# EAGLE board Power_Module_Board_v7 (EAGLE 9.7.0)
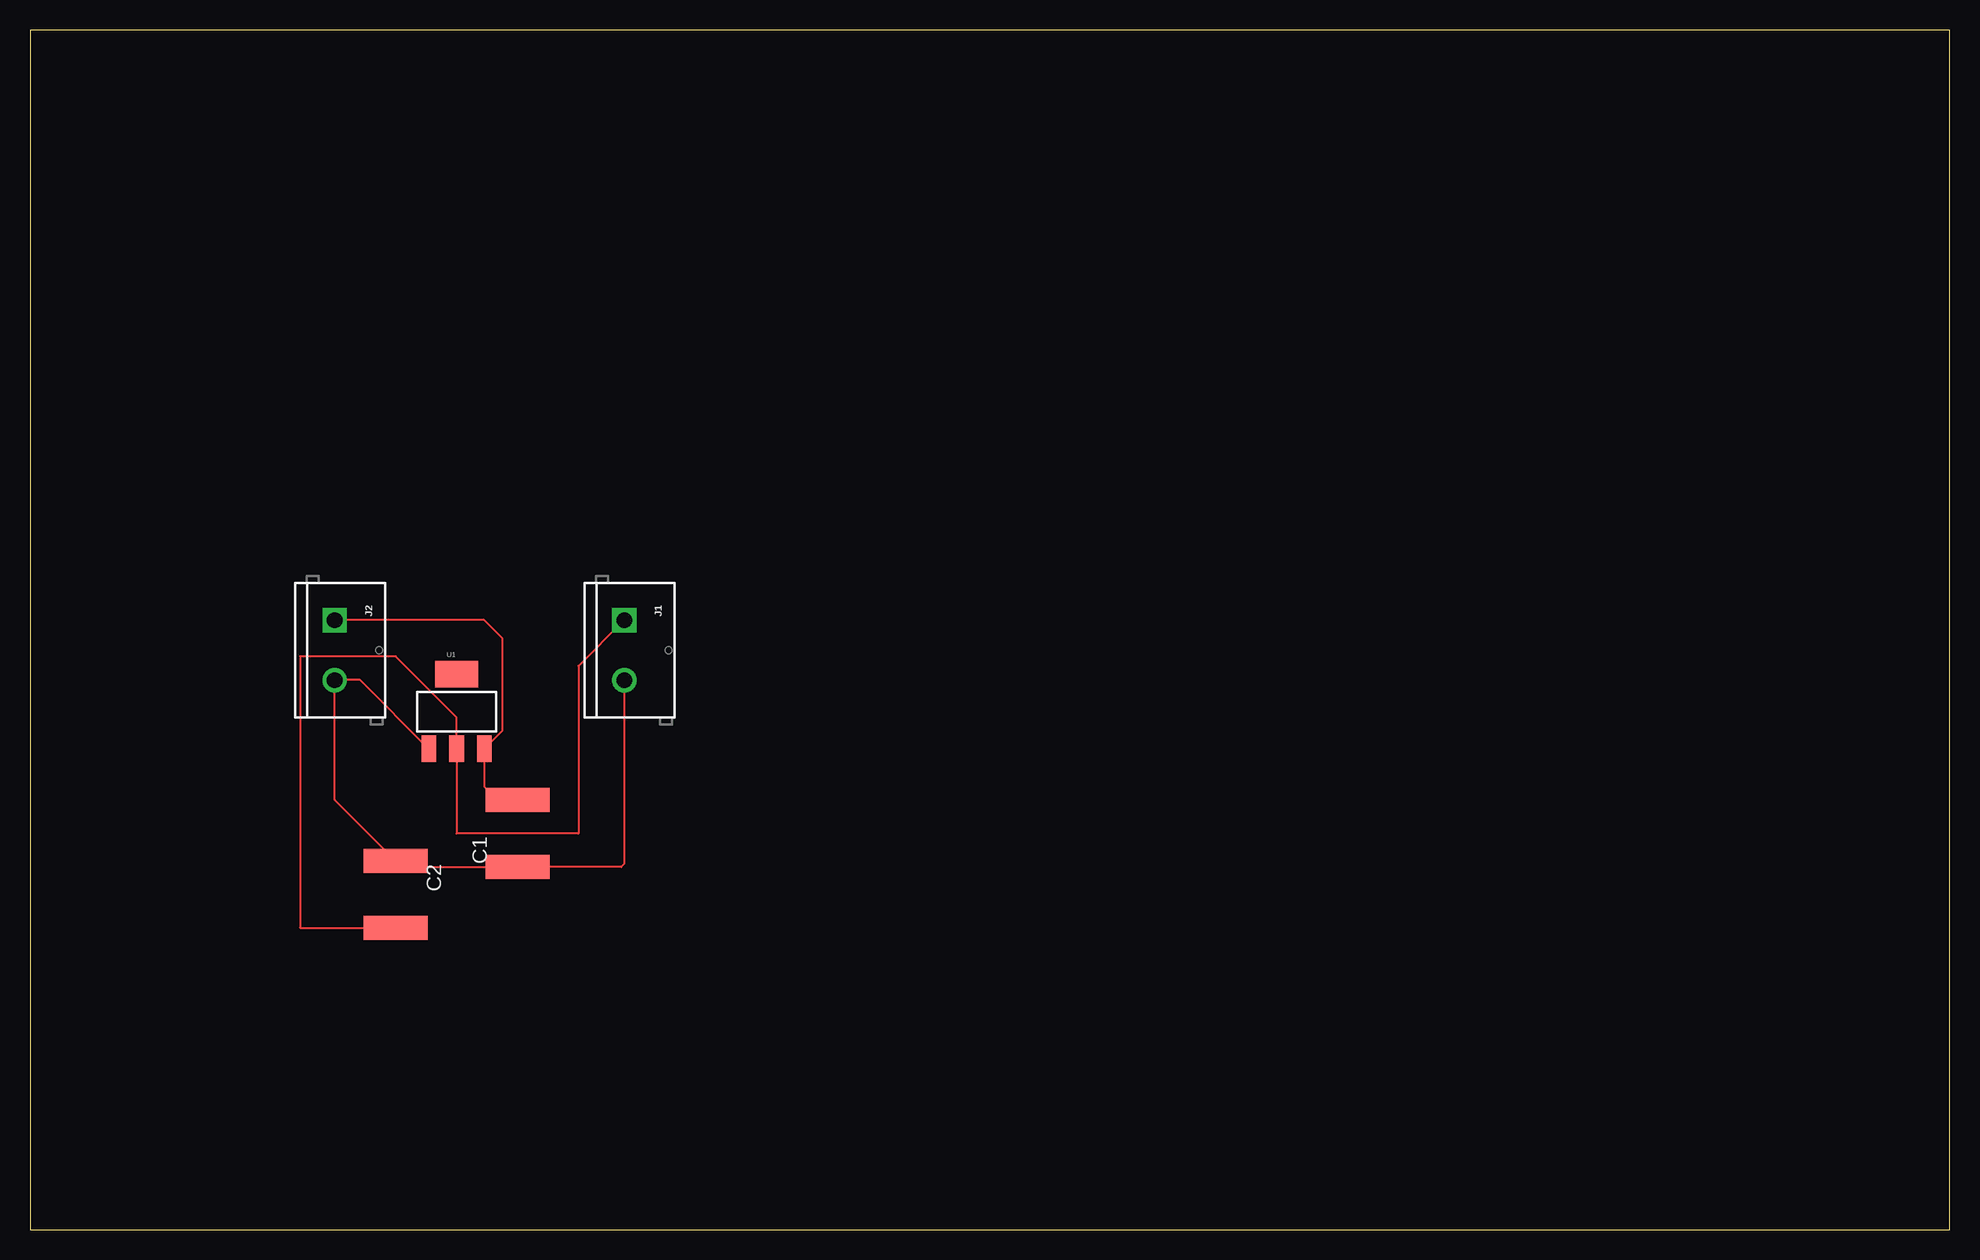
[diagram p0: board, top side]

Size 160 x 100 mm. Coordinates in mm from the lower left corner, seen from the top.
Outline: 0,0 160,0 160,100 0,100 0,0
Copper layers (1*16): Top 0.035mm / dielectric 1.5mm / Bottom 0.035mm
Design rules "default": minimum track width 6mil, minimum drill 0.35mm, track to track 6mil, track to pad 6mil, pad to pad 6mil, via to via 6mil, smd to smd 6mil, copper to edge 40mil, drill to drill 6mil, minimum pad ring 10mil, minimum via ring 8mil, stop-mask expansion 4mil, vias tented up to drill 0mil, thermal gap 10mil

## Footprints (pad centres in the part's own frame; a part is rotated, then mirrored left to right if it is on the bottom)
C2220 = smd 2.032 x 5.334: 1 -2.794,0; 2 2.794,0
SCREWTERMINAL-5MM-2 = drill 1.3 pad 2.032 square: 1 0,0 | drill 1.3 pad 2.032: 2 5,0
SOT223 = smd 1.219 x 2.235: 1 -2.311,-3.099; 2 0,-3.099; 3 2.311,-3.099 | smd 3.6 x 2.2: 4 0,3.099

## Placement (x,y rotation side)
C1  [C2220]  40.64,33.02 90 top
C2  [C2220]  30.48,27.94 270 top
J1  [SCREWTERMINAL-5MM-2]  49.53,50.8 270 top
J2  [SCREWTERMINAL-5MM-2]  25.4,50.8 270 top
U1  [SOT223]  35.56,43.18 0 top

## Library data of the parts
C1 C2 = fab
J1 J2 = SparkFun-Connectors; SF_SKU: PRT-08432
U1 = fab; PROD_ID: VREG-08170

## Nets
GND: C1.1 C2.1 J1.2 J2.2 U1.1
N$1: C1.2 J2.1 U1.3
N$4: C2.2 J1.1 U1.2

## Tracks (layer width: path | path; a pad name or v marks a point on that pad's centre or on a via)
GND
  Top 0.152: U1.1 27.53,45.8 J2.2 25.4,35.81 C2.1 30.48,30.23 C1.1 49.28,30.23 49.53,30.48 J1.2
N$1
  Top 0.152: C1.2 38.99,35.81 37.87,36.93 U1.3 39.37,41.58 39.37,49.3 37.87,50.8 J2.1
N$3  (via drill 0.35)
  other vias: 25.4,50.8
N$4
  Top 0.152: C2.2 22.5,25.15 22.5,47.78 30.48,47.78 35.56,42.7 U1.2 35.56,33.02 45.72,33.02 45.72,46.99 J1.1
N$5  (via drill 0.35)
  other vias: 25.4,45.72
N$6  (via drill 0.35)
  other vias: 49.53,50.8
N$7  (via drill 0.35)
  other vias: 49.53,45.72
